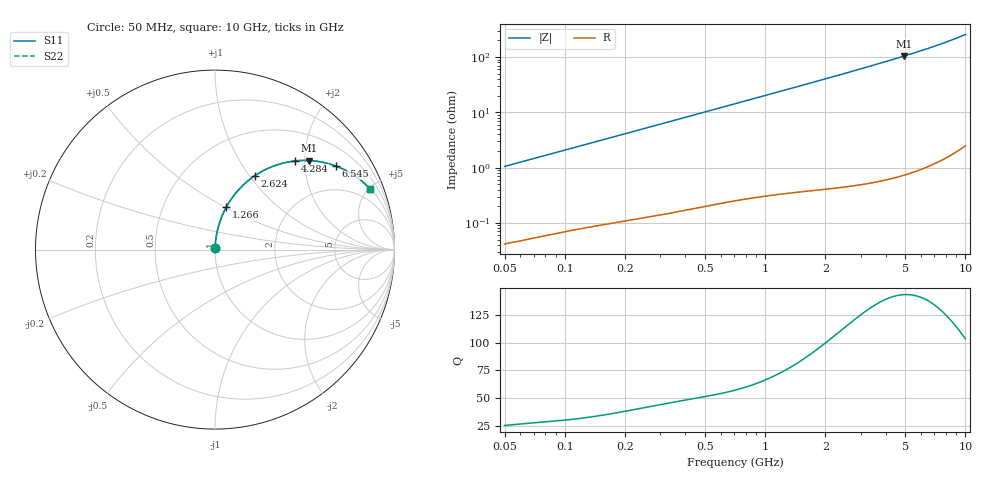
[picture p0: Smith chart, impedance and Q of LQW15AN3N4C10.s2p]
!Murata Part Number: LQW15AN3N4C10
!These Parameters are Measured in Series Mode Connection
!  o--[Z]--o
!Port1  Port2
!  o-------o
!Freq. Start=50[MHz] Stop=10[GHz], 401[Steps]
# Hz S RI R 50
!Freq.(Hz)	S 11(Real)	S 11(Imag)	S 21(Real)	S 21(Imag)	S 12(Real)	S 12(Imag)	S 22(Real)	S 22(Imag)
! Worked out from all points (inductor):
!   401 points, 50 MHz to 10 GHz, reference 50 ohm
!   read as one part in series: L = 3.33 nH near 51.34 MHz
!   highest Q = 143 at 4.956 GHz (marker M1), where L = 3.37 nH
!   S11 on the Smith chart (normalised r, x): 50 MHz: 1.00, +0.02; 1.266 GHz: 1.01, +0.51; 2.624 GHz: 1.01, +1.07; 4.284 GHz: 1.01, +1.79; 6.545 GHz: 1.02, +2.89; 10 GHz: 1.05, +5.14
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5e7  0.000526 0.0105  0.9995 -0.0105  0.9995 -0.0105  0.000526 0.0105
5.134228e7  0.000539 0.0108  0.9995 -0.0108  0.9995 -0.0108  0.000539 0.0108
1.214486e8  0.00142 0.0251  0.9986 -0.0251  0.9986 -0.0251  0.00142 0.0251
1.956524e8  0.00267 0.04  0.9973 -0.04  0.9973 -0.04  0.00267 0.04
2.949953e8  0.00497 0.0598  0.995 -0.0598  0.995 -0.0598  0.00497 0.0598
4.689809e8  0.0108 0.094  0.9892 -0.094  0.9892 -0.094  0.0108 0.094
7.071068e8  0.0224 0.1394  0.9776 -0.1394  0.9776 -0.1394  0.0224 0.1394
9.463279e8  0.0378 0.1832  0.9622 -0.1832  0.9622 -0.1832  0.0378 0.1832
1.26648e9  0.064 0.2381  0.936 -0.2381  0.936 -0.2381  0.064 0.2381
1.717543e9  0.1099 0.3073  0.8901 -0.3073  0.8901 -0.3073  0.1099 0.3073
2.122994e9  0.1581 0.36  0.8419 -0.36  0.8419 -0.36  0.1581 0.36
2.624158e9  0.2234 0.4123  0.7766 -0.4123  0.7766 -0.4123  0.2234 0.4123
3.286879e9  0.3135 0.4601  0.6865 -0.4601  0.6865 -0.4601  0.3135 0.4601
4.171863e9  0.43 0.4915  0.57 -0.4915  0.57 -0.4915  0.43 0.4915
4.283859e9  0.444 0.4933  0.556 -0.4933  0.556 -0.4933  0.444 0.4933
4.955797e9  0.5232 0.496  0.4768 -0.496  0.4768 -0.496  0.5232 0.496
5.657692e9  0.5965 0.4871  0.4035 -0.4871  0.4035 -0.4871  0.5965 0.4871
6.54512e9  0.6752 0.4647  0.3248 -0.4647  0.3248 -0.4647  0.6752 0.4647
7.37379e9  0.7359 0.437  0.2641 -0.437  0.2641 -0.437  0.7359 0.437
8.307378e9  0.7917 0.402  0.2083 -0.402  0.2083 -0.402  0.7917 0.402
9.359165e9  0.8413 0.3609  0.1587 -0.3609  0.1587 -0.3609  0.8413 0.3609
1e10  0.866 0.3358  0.134 -0.3358  0.134 -0.3358  0.866 0.3358
